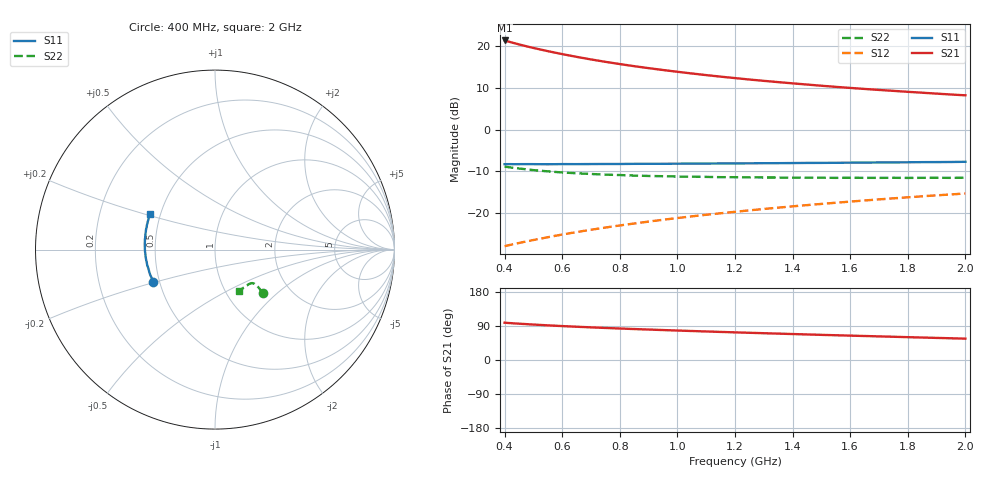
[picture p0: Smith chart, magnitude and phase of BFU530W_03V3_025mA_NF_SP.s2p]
! Filename:  P:\Prog\Test\Noise\ATS_data\Testdata_Net\06 Compressed Noise after Statistics\BFU530W_APM2013_09_A05_03p3V_025mA_NF_CM01_D.sf
! Date/Time: Tue 26/Mar/2013 18:06:06
! BFU530W_APM2013_09_A05_03p3V_1to25mA_NF_CM01_Bias9_R.sf
! Noise Parameter Data File
! BFU530W_APM2013_09_A05_03p3V_1to25mA_NF_CM01
! Date/time: Thu Mar 21 19:18:02 2013
! VAR V_out= 3.300000
! VAR I_out= 25.000000
! VAR V_in= 0.850300
! VAR I_in= 0.280650
! Device data file deembeded for feedlines and parallel
! Original file: \06 Compressed Noise after Statistics\BFU530W_APM2013_09_A05_03p3V_025mA_NF_CM01_R.sf
! Feed-files: PR019V01_070313_Feed1.s2p, PR019V01_070313_Feed2.s2p
! Parallel-file: PR019V01_070313_Par.s2p
# MHz S MA R 50
!  Freq-MHz  S11-mag  S11-arg  S21-mag  S21-arg  S12-mag  S12-arg  S22-mag  S22-arg
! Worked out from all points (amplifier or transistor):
!   37 points, 400 MHz to 2 GHz, reference 50 ohm
!   highest |S21| = 21.4 dB at 400 MHz (marker M1)
!   |S21| within 3 dB of that: start of sweep to 581 MHz
!   unconditionally stable (mu >= 1): 779 MHz to 1.979 GHz
!   at 500 MHz: K = 0.93, MSG = 23.0 dB, |S12| = -26.4 dB
!   at 1.1 GHz: K = 1.02, MAG = 15.9 dB, |S12| = -20.4 dB
!   at 2 GHz: K = 1.00, MSG = 11.8 dB, |S12| = -15.3 dB
!   lowest NFmin = 1.08 dB at 400 MHz
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400  0.3867 -152.5  11.72 98.5  0.04031 67.1  0.3614 -41.9
420  0.3871 -154.4  11.21 97.3  0.04181 67.5  0.3533 -41.8
440  0.3866 -156.3  10.74 96.3  0.04326 67.8  0.3459 -41.7
460  0.3871 -157.8  10.3 95.4  0.04478 68.2  0.34 -41.5
500  0.387 -160.9  9.53 93.5  0.04777 68.9  0.3283 -41.2
550  0.3856 -164.2  8.727 91.4  0.05162 69.7  0.3172 -40.9
600  0.3875 -167.1  8.046 89.5  0.05556 70.2  0.3076 -40.8
650  0.3871 -169.8  7.455 87.8  0.05945 70.7  0.301 -40.8
700  0.3881 -172.3  6.945 86.1  0.0634 71.2  0.2951 -40.9
750  0.3887 -174.4  6.503 84.6  0.06735 71.5  0.2898 -40.9
800  0.3886 -176.6  6.113 83.1  0.07136 71.8  0.2866 -41.4
850  0.3903 -178.6  5.769 81.7  0.07533 72.0  0.2823 -41.6
950  0.3909 178.0  5.189 79.0  0.0835 72.4  0.2776 -42.5
1050  0.393 174.7  4.715 76.5  0.09169 72.5  0.2738 -43.4
1150  0.3947 171.6  4.321 74.1  0.09987 72.5  0.2704 -44.7
1200  0.3948 170.2  4.153 72.9  0.1041 72.5  0.2701 -45.5
1250  0.3958 168.8  3.992 71.8  0.1082 72.4  0.2685 -46.1
1350  0.3977 166.4  3.716 69.6  0.1167 72.2  0.2677 -47.7
1500  0.4006 162.5  3.364 66.3  0.1293 71.7  0.2663 -50.4
1650  0.4037 159.0  3.078 63.3  0.1421 71.2  0.2652 -53.0
1750  0.4061 156.8  2.92 61.3  0.1507 70.7  0.2656 -54.9
2000  0.4129 151.4  2.582 56.4  0.1723 69.4  0.2663 -60.0
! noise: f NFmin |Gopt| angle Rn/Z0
400  1.082  0.3632  -170.4  0.0642
460  1.095  0.3643  -171  0.0646
600  1.107  0.3694  -167.2  0.0671
800  1.16  0.3892  -163.4  0.065
1000  1.194  0.3961  -158.1  0.07
1200  1.279  0.3988  -155  0.0752
1400  1.285  0.4166  -149.3  0.0825
1600  1.272  0.4693  -146.1  0.0776
1800  1.35  0.4431  -140.5  0.1013
2000  1.416  0.4581  -136.1  0.113
